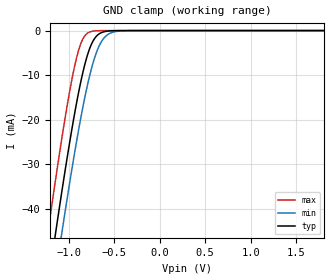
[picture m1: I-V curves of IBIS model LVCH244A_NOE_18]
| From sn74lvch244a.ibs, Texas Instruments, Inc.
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[Model]   LVCH244A_NOE_18
Model_type  Input
Vinl=0.5775
Vinh=1.2675
| variable   typ   min   max
C_comp   3.37pF   3.10pF   3.92pF
[Temperature Range]   40   100   -40
| Ambient temperature   25   85   -40
[Voltage range]   1.8   1.65   1.95
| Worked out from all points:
|   GND clamp passes 1 mA (typ) near -0.68 V on its own axis
[GND Clamp]
| LVCH244A_NOE_18
|   Voltage   I(typ)   I(min)   I(max)
-5.5V     -731.8mA   -738.6mA   -723.7mA
-1.225V   -57.15mA   -66.48mA   -45.16mA
-1.145V   -45.9mA    -55.24mA   -33.86mA
-1.08V    -37.05mA   -46.34mA   -25.08mA
-1.06V    -34.39mA   -43.66mA   -22.48mA
-945mV    -20.02mA   -28.9mA    -9.143mA
-855mV    -10.53mA   -18.51mA   -2.421mA
-735mV    -2.503mA   -7.547mA   -134.2uA
-660mV    -683.9uA   -3.283mA   -17.65uA
-580mV    -143.9uA   -1.059mA   -1.991uA
-330mV    -907.1nA   -16.53uA   -2.162nA
1.8V      1.113nA    59.61nA    5.028pA
